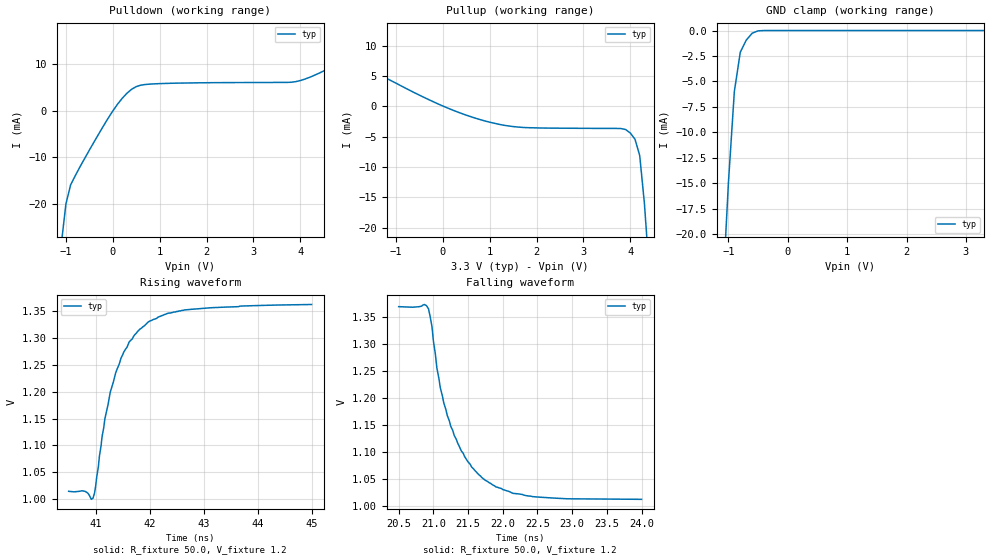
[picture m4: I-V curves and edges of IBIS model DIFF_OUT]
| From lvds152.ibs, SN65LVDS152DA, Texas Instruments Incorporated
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|   Cascade Driver Output  MODEL
[Model]   DIFF_OUT
Model_type   3-state
| Signals   CO+,CO-
Vmeas = 1.2V   |Reference voltage for timing measurements
Cref = 5pF   |Timing specification test load capacitance value
Rref = 50   |Note: 50 Ohm load; single ended configuration
Vref = 1.18V   |Timing specification test load voltage
| variable   typ   min   max
C_comp   1.0pF   NA   NA
|   typ   min   max
[Temperature Range]   25.0   NA   NA
[Voltage range]   3.3V   3.0V   3.6V
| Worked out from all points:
|   slope of the pulldown table from 0 to 0.495 V, typ, clamps not added: 94.8 ohm
|   slope of the pullup table from 0 to 0.495 V, typ, clamps not added: 330 ohm
|   GND clamp passes 1 mA (typ) near -0.70 V on its own axis
|   rising waveform, R_fixture 50.0, V_fixture 1.2: 20-80 % time 546ps typ, NA min, NA max; typ from 1.01 V to 1.36 V
|   falling waveform, R_fixture 50.0, V_fixture 1.2: 20-80 % time 480ps typ, NA min, NA max; typ from 1.37 V to 1.01 V
[Pulldown]
|   Voltage   I(typ)   I(min)   I(max)
-3.3V     -317mA     NA         NA
-1.1V     -28.9mA    NA         NA
-1V       -20.1mA    NA         NA
-900mV    -16mA      NA         NA
-800mV    -14mA      NA         NA
0V        -81.9uA    NA         NA
300mV     3.72mA     NA         NA
500mV     5.17mA     NA         NA
1V        5.81mA     NA         NA
3.9V      6.23mA     NA         NA
4.3V      7.6mA      NA         NA
6.6V      17.9mA     NA         NA
[Pullup]
|   Voltage   I(typ)   I(min)   I(max)
| Note that the[Pullup]voltage table is referenced to Vcc
| and is calculated using Vtable=Vcc - Vmeasured.
-3.3V     13mA       NA         NA
-500mV    1.87mA     NA         NA
700mV     -1.94mA    NA         NA
1.2V      -2.94mA    NA         NA
1.7V      -3.45mA    NA         NA
3.9V      -3.8mA     NA         NA
4V        -4.38mA    NA         NA
4.1V      -5.4mA     NA         NA
4.2V      -8.07mA    NA         NA
4.3V      -15.9mA    NA         NA
4.4V      -26.8mA    NA         NA
6.6V      -317mA     NA         NA
[GND_clamp]
|   Voltage   I(typ)   I(min)   I(max)
| Outputs in High Impedance (off)
-3.3V     -317mA     NA         NA
-1.1V     -26.3mA    NA         NA
-1V       -15mA      NA         NA
-900mV    -6mA       NA         NA
-800mV    -2.13mA    NA         NA
-700mV    -949uA     NA         NA
-600mV    -264uA     NA         NA
-500mV    -32.5uA    NA         NA
-400mV    -2.47uA    NA         NA
3.3V      246pA      NA         NA
[POWER_clamp]
|   Voltage   I(typ)   I(min)   I(max)
| Note that the [POWER_clamp] voltage table is referenced to Vcc
| and is calculated using Vtable = Vcc - Vmeasured.
| Outputs in Tri-state.
-3.3V     0A         NA         NA
0V        0A         NA         NA
[Ramp]
|   typ   min   max
dV/dt_r   0.209/610ps   NA   NA
dV/dt_f   0.213/490ps   NA   NA
R_load = 50ohm  | Note: The measurement is single-ended with 50ohm
|   to ground.
[Rising Waveform]
R_fixture = 50.0
V_fixture = 1.2
C_fixture = 0p
L_fixture = 0n
|   V(typ)   V(min)   V(max)
40.5ns    1.014V     NA         NA
40.8ns    1.014V     NA         NA
40.95ns   1.001V     NA         NA
41ns      1.024V     NA         NA
41.17ns   1.149V     NA         NA
41.37ns   1.235V     NA         NA
41.62ns   1.293V     NA         NA
41.97ns   1.33V      NA         NA
42.65ns   1.353V     NA         NA
45ns      1.363V     NA         NA
[Falling Waveform]
R_fixture = 50.0
V_fixture = 1.2
C_fixture = 0p
L_fixture = 0n
|   V(typ)   V(min)   V(max)
20.5ns    1.369V     NA         NA
20.93ns   1.365V     NA         NA
20.98ns   1.332V     NA         NA
21.05ns   1.256V     NA         NA
21.1ns    1.219V     NA         NA
21.2ns    1.168V     NA         NA
21.4ns    1.103V     NA         NA
21.7ns    1.053V     NA         NA
22.43ns   1.018V     NA         NA
24ns      1.013V     NA         NA
